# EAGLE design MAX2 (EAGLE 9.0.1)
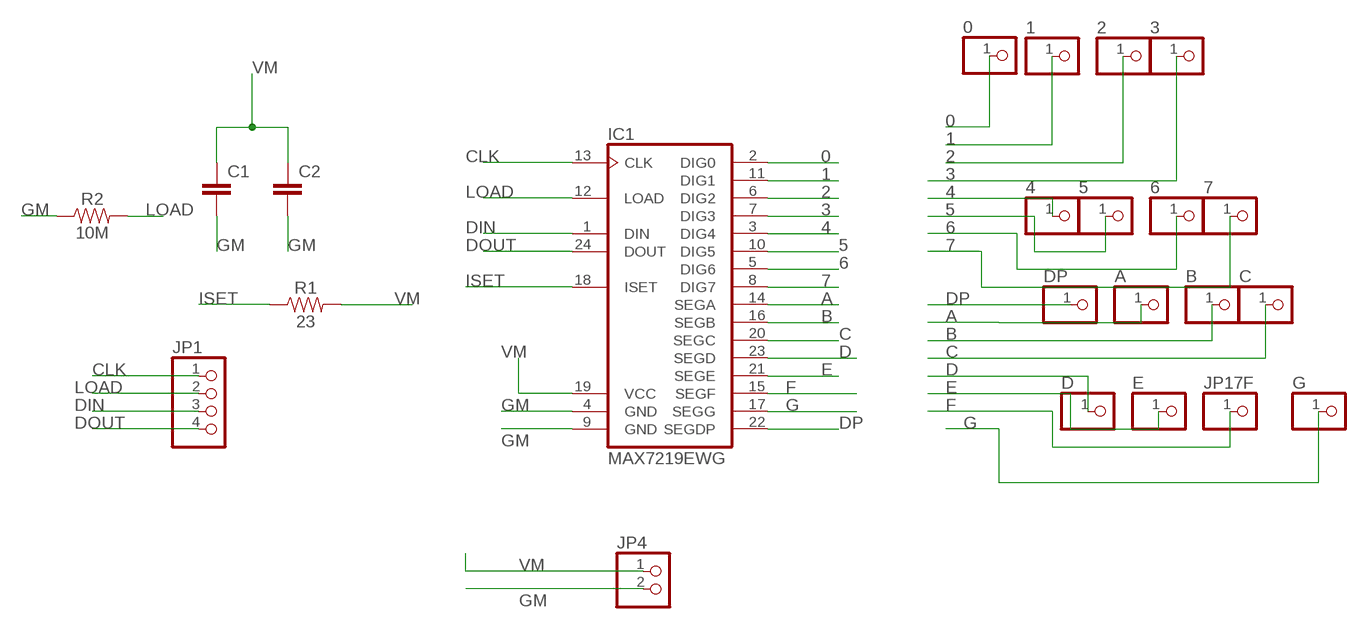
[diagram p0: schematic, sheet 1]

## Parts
0  PINHD-1X1  [1X01]
1  PINHD-1X1  [1X01]
2  PINHD-1X1  [1X01]
3  PINHD-1X1  [1X01]
4  PINHD-1X1  [1X01]
5  PINHD-1X1  [1X01]
6  PINHD-1X1  [1X01]
7  PINHD-1X1  [1X01]
A  PINHD-1X1  [1X01]
B  PINHD-1X1  [1X01]
C  PINHD-1X1  [1X01]
C1  C2,5-3  [C2.5-3]
C2  C5/7.2  [C5B7.2]
D  PINHD-1X1  [1X01]
DP  PINHD-1X1  [1X01]
E  PINHD-1X1  [1X01]
G  PINHD-1X1  [1X01]
IC1  MAX7219EWG  [SO24W]
JP1  PINHD-1X4/90  [1X04/90]
JP4  PINHD-1X2  [1X02]
JP17F  PINHD-1X1  [1X01]
R1  23  10MOHM-HORIZ-1/4W-5%  [AXIAL-0.3]
R2  10M  10MOHM-HORIZ-1/4W-5%  [AXIAL-0.3]

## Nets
0: 0.1 IC1.2(DIG0)
1: 1.1 IC1.11(DIG1)
2: 2.1 IC1.6(DIG2)
3: 3.1 IC1.7(DIG3)
4: 4.1 IC1.3(DIG4)
5: 5.1 IC1.10(DIG5)
6: 6.1 IC1.5(DIG6)
7: 7.1 IC1.8(DIG7)
A: A.1 IC1.14(SEGA)
B: B.1 IC1.16(SEGB)
C: C.1 IC1.20(SEGC)
CLK: IC1.13(CLK) JP1.1
D: D.1 IC1.23(SEGD)
DIN: IC1.1(DIN) JP1.3
DOUT: IC1.24(DOUT) JP1.4
DP: DP.1 IC1.22(SEGDP)
E: E.1 IC1.21(SEGE)
F: IC1.15(SEGF) JP17F.1
G: G.1 IC1.17(SEGG)
GM: C1.2 C2.2 IC1.4(GND) IC1.9(GND) JP4.2 R2.P$1
ISET: IC1.18(ISET) R1.P$1
LOAD: IC1.12(LOAD) JP1.2 R2.P$2
VM: C1.1 C2.1 IC1.19(VCC) JP4.1 R1.P$2

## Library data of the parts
0 1-7 A B C D DP E G JP17F = pinhead:PINHD-1X1: PIN HEADER
C1 C2 = capacitor-wima:C: CAPACITOR
IC1 = maxim-8:MAX7219*: Serially Interfaced, 8-Digit LED Display Drivers
JP1 = DC_LOAD_AU:PINHD-1X4: PIN HEADER
JP4 = pinhead:PINHD-1X2: PIN HEADER
R1 = SparkFun-Resistors:10MOHM: RES-09327; PROD_ID: RES-09327; VALUE: 10M
R2 = SparkFun-Resistors:10MOHM: RES-09327; PROD_ID: RES-09327

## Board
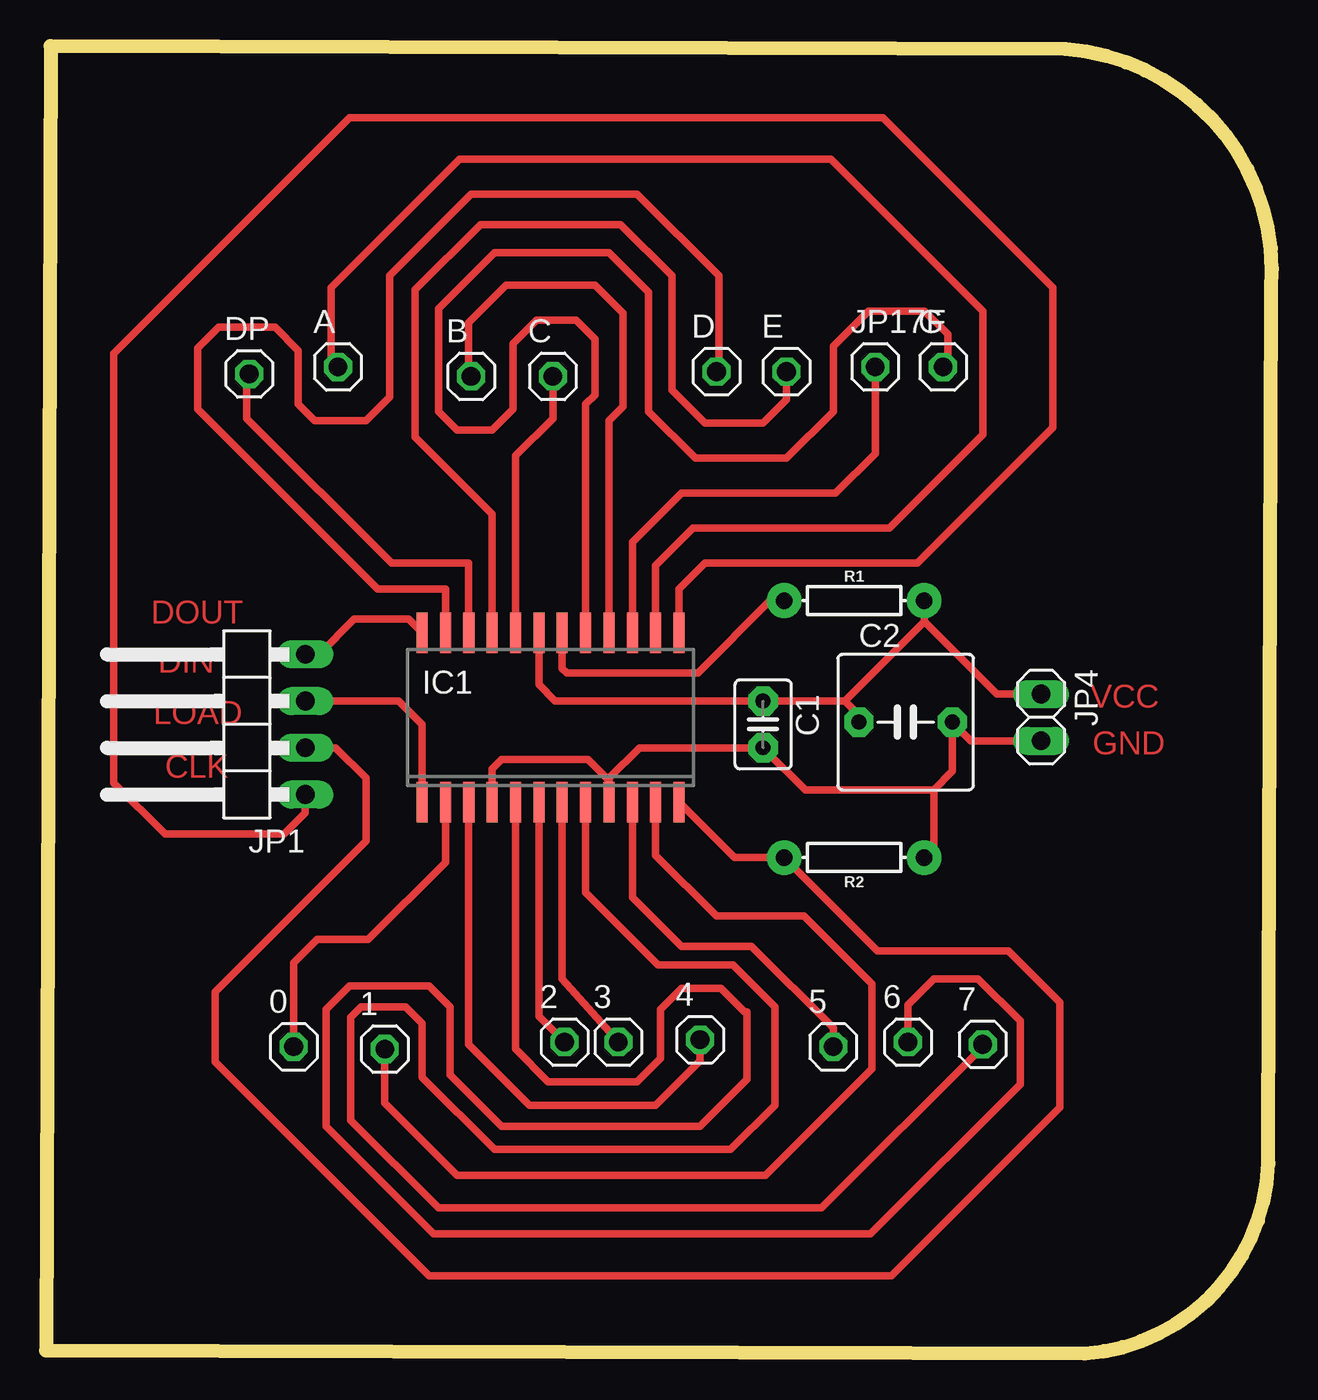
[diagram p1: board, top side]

Size 66.65 x 71.08 mm. Coordinates in mm from the lower left corner, seen from the top.
Outline: 0,0.17 56.47,0 arc90 66.44,11.36 66.61,57.83 arc90 55.44,70.91 0.25,71.08 0,0.17
Copper layers (1*16): Top 0.035mm / dielectric 1.5mm / Bottom 0.035mm
Design rules "default *": minimum track width 18mil, minimum drill 0.35mm, track to track 16mil, track to pad 16mil, pad to pad 16mil, via to via 16mil, smd to smd 16mil, copper to edge 40mil, drill to drill 6mil, minimum pad ring 10mil, minimum via ring 8mil, stop-mask expansion 4mil, vias tented up to drill 0mil, thermal gap 10mil

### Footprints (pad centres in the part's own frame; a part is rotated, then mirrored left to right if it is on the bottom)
1X01 = drill 1.016 octagon: 1 0,0
C2.5-3 = drill 0.813 pad 1.6 octagon: 1 -1.27,0; 2 1.27,0
C5B7.2 = drill 0.813 pad 1.6 octagon: 1 -2.54,0; 2 2.54,0
SO24W = smd 0.6 x 2.2: 1 -6.985,-4.6; 2 -5.715,-4.6; 3 -4.445,-4.6; 4 -3.175,-4.6; 5 -1.905,-4.6; 6 -0.635,-4.6; 7 0.635,-4.6; 8 1.905,-4.6; 9 3.175,-4.6; 10 4.445,-4.6; 11 5.715,-4.6; 12 6.985,-4.6; 13 6.985,4.6; 14 5.715,4.6; 15 4.445,4.6; 16 3.175,4.6; 17 1.905,4.6; 18 0.635,4.6; 19 -0.635,4.6; 20 -1.905,4.6; 21 -3.175,4.6; 22 -4.445,4.6; 23 -5.715,4.6; 24 -6.985,4.6
1X04/90 = drill 1.016 long: 1 -3.81,-3.81; 2 -1.27,-3.81; 3 1.27,-3.81; 4 3.81,-3.81
1X02 = drill 1.016 long: 1 -1.27,0; 2 1.27,0
AXIAL-0.3 = drill 0.9 pad 1.88: P$1 -3.81,0; P$2 3.81,0

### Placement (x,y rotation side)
0  13.46,16.68 0 top
1  18.41,16.55 0 top
2  28.19,16.93 0 top
3  31.12,16.93 0 top
4  35.56,17.06 0 top
5  42.8,16.68 0 top
6  46.86,16.93 0 top
7  50.93,16.8 0 top
A  15.88,53.63 0 top
B  23.11,53.12 0 top
C  27.56,53.12 0 top
C1  38.99,34.2 270 top
C2  46.74,34.33 0 top
D  36.45,53.38 0 top
DP  11.05,53.25 0 top
E  40.26,53.38 0 top
G  48.77,53.63 0 top
IC1  27.43,34.58 0 top
JP1  10.29,34.2 90 top
JP4  54.1,34.58 270 top
JP17F  45.09,53.63 0 top
R1  43.94,40.93 0 top
R2  43.94,26.96 180 top

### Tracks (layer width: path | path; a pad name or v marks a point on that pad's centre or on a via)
0
  Top 0.406: IC1.2 21.72,26.71 17.53,22.52 14.73,22.52 13.46,21.25 0.1
1
  Top 0.406: IC1.11 33.15,27.09 36.45,23.79 41.21,23.79 44.9,20.1 44.9,15.47 39.12,9.69 22.35,9.69 18.41,13.63 1.1
2
  Top 0.406: IC1.6 26.8,18.33 2.1
3
  Top 0.406: IC1.7 28.07,20.36 3.1
4
  Top 0.406: 4.1 35.56,15.91 33.15,13.5 26.29,13.5 22.99,16.8 IC1.3
5
  Top 0.406: 31.88,28.87 IC1.10 31.88,24.8 34.54,22.14 38.35,22.14 42.8,17.69 5.1
6
  Top 0.406: 6.1 46.86,18.96 48.26,20.36 50.67,20.36 52.96,18.07 52.96,14.64 44.83,6.52 21.08,6.52 15.24,12.36 15.24,18.71 16.51,19.98 20.83,19.98 21.97,18.83 21.97,15.15 24.77,12.36 35.56,12.36 38.1,14.9 38.1,18.58 37.97,18.58 36.7,19.85 34.54,19.85 33.4,18.71 33.4,16.04 32.13,14.77 27.3,14.77 25.53,16.55 IC1.5
7
  Top 0.406: 29.34,28.99 IC1.8 29.34,25.06 33.27,21.12 37.34,21.12 39.62,18.83 39.62,13.5 37.21,11.09 24.38,11.09 20.45,15.02 20.45,17.95 19.56,18.83 17.14,18.83 16.57,18.26 16.57,12.67 21.34,7.91 42.16,7.91 50.93,16.68 7.1
A
  Top 0.406: IC1.14 33.15,42.84 35.18,44.87 45.85,44.87 50.93,49.95 50.93,56.68 42.67,64.94 22.48,64.94 15.49,57.95 15.49,54.01 A.1
B
  Top 0.406: IC1.16 30.61,50.71 31.37,51.47 31.37,56.55 29.84,58.08 25.02,58.08 22.99,56.05 22.99,53.25 B.1
C
  Top 0.406: C.1 27.43,53 27.56,52.87 27.56,50.84 25.53,48.81 IC1.20
CLK
  Top 0.406: IC1.13 34.42,41.57 35.81,42.96 47.37,42.96 54.74,50.33 54.74,57.95 45.49,67.2 16.51,67.2 3.68,54.37 3.68,31.03 6.48,28.23 12.95,28.23 14.1,29.38 JP1.1 13.97,30.26
D
  Top 0.406: IC1.23 21.72,41.57 18.03,41.57 8.26,51.35 8.26,54.65 9.4,55.79 12.45,55.79 13.72,54.52 13.72,51.6 14.61,50.71 17.4,50.71 18.67,51.98 18.67,58.59 23.11,63.03 32.13,63.03 36.58,58.59 36.58,53.51 D.1
DIN
  Top 0.406: IC1.1 20.45,34.2 19.18,35.47 JP1.3
DOUT
  Top 0.406: IC1.24 19.71,39.92 16.76,39.92 14.86,38.01 JP1.4
DP
  Top 0.406: IC1.22 22.99,42.96 18.8,42.96 10.92,50.84 10.92,53.12 DP.1
E
  Top 0.406: IC1.21 24.26,45.63 20.07,49.82 20.07,57.82 23.62,61.38 31.24,61.38 34.04,58.59 34.04,52.36 35.81,50.58 38.99,50.58 40.26,51.85 E.1
F
  Top 0.406: IC1.15 31.88,44.11 34.54,46.77 42.93,46.77 45.09,48.93 JP17F.1
G
  Top 0.406: IC1.17 29.34,51.6 29.84,52.11 29.84,55.16 28.83,56.17 26.67,56.17 25.4,54.9 25.4,51.35 24.26,50.2 22.35,50.2 21.34,51.22 21.34,56.81 24.38,59.86 30.61,59.86 32.77,57.7 32.77,51.22 35.31,48.68 40.26,48.68 42.8,51.22 42.8,54.78 44.7,56.68 47.75,56.68 49.02,55.41 49.02,53.89 G.1
GM
  Top 0.406: IC1.4 24.26,31.79 24.77,32.3 29.46,32.3 30.61,31.15 IC1.9 30.61,31.28 32.26,32.93 C1.2 41.27,30.65 48.26,30.65 | 48.26,30.65 49.28,31.66 C2.2 50.29,33.31 JP4.2 | 48.26,30.65 48.26,27.47 R2.P$1
ISET
  Top 0.406: IC1.18 28.07,37.25 28.32,37 35.43,37 39.37,40.93 R1.P$1
LOAD
  Top 0.406: IC1.12 37.44,26.96 R2.P$2 45.21,21.88 52.32,21.88 55.12,19.09 55.12,18.96 55.12,18.83 55.12,13.37 45.97,4.23 20.83,4.23 9.21,15.85 9.21,19.66 17.4,27.85 17.4,31.28 15.75,32.93 JP1.2
VM
  Top 0.406: IC1.19 26.8,36.36 27.69,35.47 C1.1 43.43,35.47 | 43.43,35.47 44.2,34.71 C2.1 | 43.43,35.47 47.75,39.79 | 47.75,39.79 R1.P$2 | 47.75,39.79 51.69,35.85 JP4.1

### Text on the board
Top: DOUT | DIN | VCC | LOAD | GND | CLK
